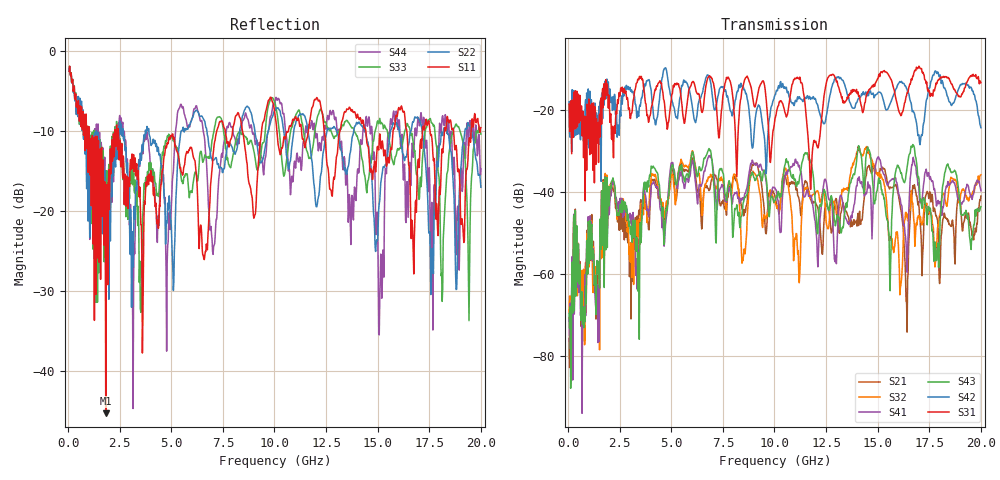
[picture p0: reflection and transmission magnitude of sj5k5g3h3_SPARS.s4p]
! FILE: E:\users\goganessyan\GBX_Backplane\FR408_backplane\1m_OUTBOUND_NEXT\sj5k5g3h3_SPARS.s4p
# MHZ S RI R 50.00
! FREQ  S11  S12  S13  S14
!  S21  S22  S23  S24
!  S31  S32  S33  S34
!  S41  S42  S43  S44
!  REAL  IMAG  REAL  IMAG  REAL  IMAG  REAL  IMAG
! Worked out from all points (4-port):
!   799 points, 50 MHz to 20 GHz, reference 50 ohm
!   strongest paths, dB at 50 MHz, 5.025 GHz, 10.03 GHz, 15.03 GHz, 20 GHz:
!     S31: -18.7, -16.3, -22.2, -12.3, -13.4
!     S42: -18.1, -17.7, -16.4, -15.8, -24.4
!     S43: -69.6, -33.8, -42.1, -37.5, -43.6
!     S41: -70.6, -33.1, -39.1, -31.5, -39.7
!     S32: -69.2, -35.8, -42.3, -36.1, -35.8
!     S21: -75.7, -34.4, -41.0, -35.5, -41.0
!   lowest |S11| = -45.3 dB at 1.825 GHz (marker M1), VSWR 1.01, Z = 50.5 - j0.116 ohm
!   |S11| at or under -10 dB: 1.027 GHz to 2.273 GHz (1.246 GHz wide, 75.5 % of centre); 2.432 GHz to 7.202 GHz (4.77 GHz wide, 99 % of centre); 14.43 GHz to 15.75 GHz (1.319 GHz wide, 8.74 % of centre)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
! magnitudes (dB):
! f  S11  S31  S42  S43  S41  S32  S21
! 50 MHz  -2.5  -18.7  -18.1  -69.6  -70.6  -69.2  -75.7
! 1.825 GHz  -45.3  -12.7  -17.4  -54.1  -49.9  -50.6  -52.9
! 10.53 GHz  -11.0  -20.9  -14.9  -33.2  -36.3  -34.2  -36.6
! 11.18 GHz  -8.5  -12.5  -17.3  -38.0  -33.9  -59.3  -41.4
! 14.45 GHz  -10.7  -16.6  -16.4  -30.9  -40.5  -29.1  -36.1
! 16.12 GHz  -7.0  -21.5  -13.3  -35.5  -43.0  -62.5  -44.5
! 20 GHz  -9.6  -13.4  -24.4  -43.6  -39.7  -35.8  -41.0
